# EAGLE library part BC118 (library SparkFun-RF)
Blue Creation BC118 Bluetooth 4.0 Audio Module BC118 consists of a Bluetooth Smart (Bluetooth 4.0) radio, a microprocessor running an embedded protocol stack. The module is controlled by high level UART instructions or GPIOs. B118 supports UART and I2C Transparent mode for cable replacement, standard/custom profiles, central and peripheral modes. It can connect to any Android, iOS or Windows Mobile Smartphone that is Bluetooth smart capable. The firmware can be upgraded using an App provided by BlueCreation. BC118 can run standalone, with a host processor or controlled by an App. Datasheet SparkFun Products: BLE Mate 2 (WRL-13019)
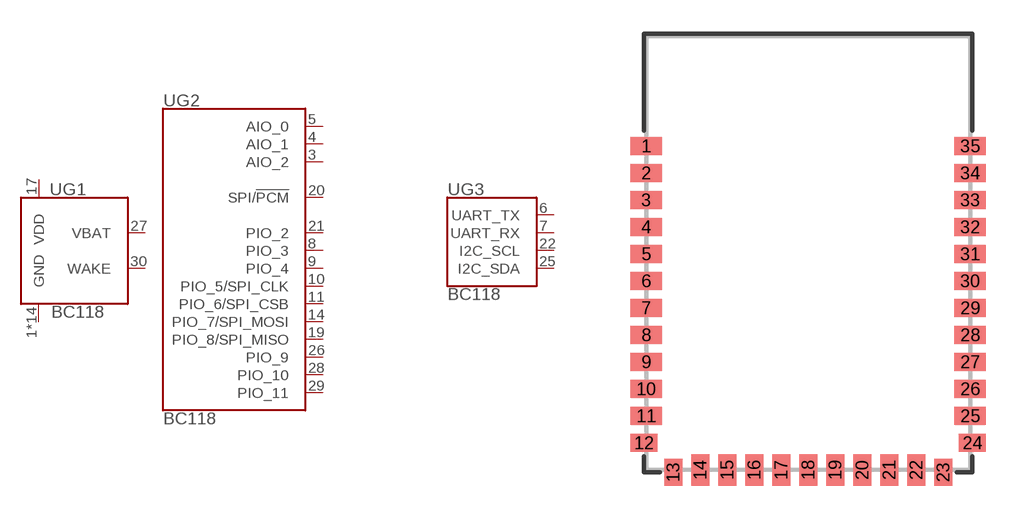
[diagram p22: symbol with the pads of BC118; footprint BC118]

Designator prefix U; gates G1=BC118_POWER G2=BC118_PIO G3=BC118_COMMS

## BC118 (PROD_ID: WRL-12203; VALUE: BC118)  [BC118]
1  G1:GND
2  G1:GND
3  G2:AIO_2
4  G2:AIO_1
5  G2:AIO_0
6  G3:UART_TX
7  G3:UART_RX
8  G2:PIO_3
9  G2:PIO_4
10  G2:PIO_5/SPI_CLK
11  G2:PIO_6/SPI_CSB
12  G1:GND
13  G1:GND
14  G2:PIO_7/SPI_MOSI
15  G1:GND
16  G1:GND
17  G1:VDD
18  G1:GND
19  G2:PIO_8/SPI_MISO
20  G2:SPI/!PCM
21  G2:PIO_2
22  G3:I2C_SCL
23  G1:GND
24  G1:GND
25  G3:I2C_SDA
26  G2:PIO_9
27  G1:VBAT
28  G2:PIO_10
29  G2:PIO_11
30  G1:WAKE
31  G1:GND
32  G1:GND
33  G1:GND
34  G1:GND
35  G1:GND

## Footprint BC118 (pad centres in mm)
Blue Creation BC118 Bluetooth 4.0 Audio Module 14.4x19.3mm Datasheet
smd 1.4 x 0.8: 1 -7.2,4.75; 2 -7.2,3.55; 3 -7.2,2.35; 4 -7.2,1.15; 5 -7.2,-0.05; 6 -7.2,-1.25; 7 -7.2,-2.45; 8 -7.2,-3.65; 9 -7.2,-4.85; 10 -7.2,-6.05; 11 -7.2,-7.25; 25 7.2,-7.25; 26 7.2,-6.05; 27 7.2,-4.85; 28 7.2,-3.65; 29 7.2,-2.45; 30 7.2,-1.25; 31 7.2,-0.05; 32 7.2,1.15; 33 7.2,2.35; 34 7.2,3.55; 35 7.2,4.75
smd 1.2 x 0.8: 12 -7.3,-8.45; 24 7.3,-8.45
smd 0.8 x 1.2: 13 -6,-9.75; 23 6,-9.75
smd 0.8 x 1.4: 14 -4.8,-9.65; 15 -3.6,-9.65; 16 -2.4,-9.65; 17 -1.2,-9.65; 18 0,-9.65; 19 1.2,-9.65; 20 2.4,-9.65; 21 3.6,-9.65; 22 4.8,-9.65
